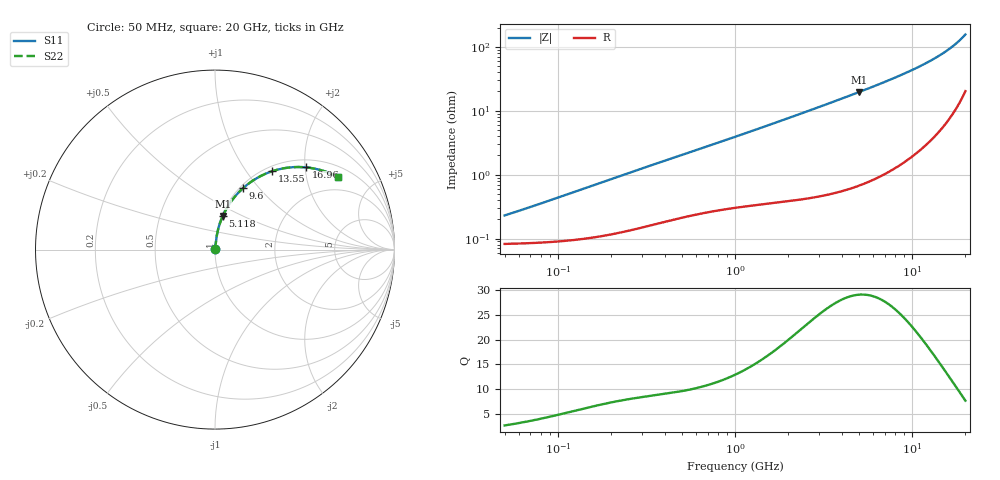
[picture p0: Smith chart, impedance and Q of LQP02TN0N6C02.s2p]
!Murata Part Number: LQP02TN0N6C02
!These Parameters are Measured in Series Mode Connection
!  o--[Z]--o
!Port1  Port2
!  o-------o
!Freq. Start=50[MHz] Stop=20[GHz], 401[Steps]
# Hz S RI R 50
!Freq.(Hz) S11(Real) S11(Imag) S21(Real) S21(Imag) S12(Real) S12(Imag) S22(Real) S22(Imag)
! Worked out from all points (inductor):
!   401 points, 50 MHz to 20 GHz, reference 50 ohm
!   read as one part in series: L = 681 pH near 58.96 MHz
!   highest Q = 29.1 at 5.041 GHz (marker M1), where L = 621 pH
!   S11 on the Smith chart (normalised r, x): 50 MHz: 1.00, +0.00; 5.118 GHz: 1.01, +0.40; 9.6 GHz: 1.04, +0.82; 13.55 GHz: 1.08, +1.34; 16.96 GHz: 1.18, +2.03; 20 GHz: 1.41, +3.10
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5e7  0.000826 0.00214  0.9992 -0.00214  0.9992 -0.00214  0.000826 0.00214
6.951576e7  0.000855 0.00297  0.9991 -0.00297  0.9991 -0.00297  0.000855 0.00297
1.364002e8  0.00101 0.00579  0.999 -0.00579  0.999 -0.00579  0.00101 0.00579
3.721004e8  0.00196 0.0152  0.998 -0.0152  0.998 -0.0152  0.00196 0.0152
1e9  0.0045 0.0386  0.9955 -0.0386  0.9955 -0.0386  0.0045 0.0386
1.714689e9  0.00787 0.0649  0.9921 -0.0649  0.9921 -0.0649  0.00787 0.0649
2.728004e9  0.015 0.1023  0.985 -0.1023  0.985 -0.1023  0.015 0.1023
3.736399e9  0.0251 0.1394  0.9749 -0.1394  0.9749 -0.1394  0.0251 0.1394
5.041459e9  0.0432 0.1869  0.9568 -0.1869  0.9568 -0.1869  0.0432 0.1869
5.117541e9  0.0445 0.1897  0.9555 -0.1897  0.9555 -0.1897  0.0445 0.1897
6.217679e9  0.0646 0.2289  0.9354 -0.2289  0.9354 -0.2289  0.0646 0.2289
7.442007e9  0.0921 0.2713  0.9079 -0.2713  0.9079 -0.2713  0.0921 0.2713
8.516016e9  0.121 0.307  0.879 -0.307  0.879 -0.307  0.121 0.307
9.600142e9  0.1549 0.3411  0.8451 -0.3411  0.8451 -0.3411  0.1549 0.3411
1.149051e10  0.2258 0.3938  0.7742 -0.3938  0.7742 -0.3938  0.2258 0.3938
1.257102e10  0.2731 0.4187  0.7269 -0.4187  0.7269 -0.4187  0.2731 0.4187
1.354865e10  0.32 0.4371  0.68 -0.4371  0.68 -0.4371  0.32 0.4371
1.527346e10  0.4113 0.4571  0.5887 -0.4571  0.5887 -0.4571  0.4113 0.4571
1.696185e10  0.5086 0.458  0.4914 -0.458  0.4914 -0.458  0.5086 0.458
1.828096e10  0.587 0.4435  0.413 -0.4435  0.413 -0.4435  0.587 0.4435
1.940974e10  0.6533 0.4196  0.3467 -0.4196  0.3467 -0.4196  0.6533 0.4196
2e10  0.6869 0.4029  0.3131 -0.4029  0.3131 -0.4029  0.6869 0.4029
